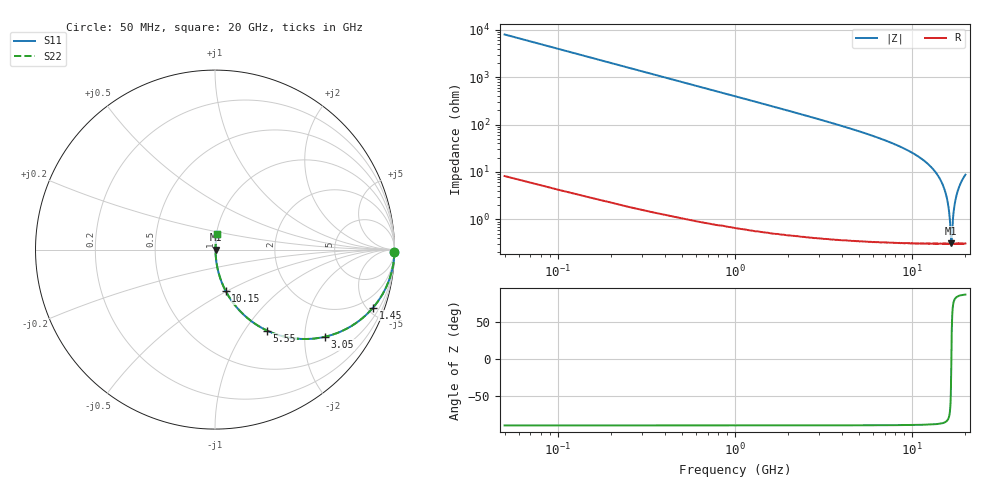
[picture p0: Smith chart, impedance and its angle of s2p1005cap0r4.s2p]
!	AVX	Thin	Film	Operation
!	Date:	March 2012
!	Description: Ultra-Miniature 01005 Size ACCU - P® Thin Film RF / Microwave Capacitor
!	Part Number:  C005YJ0R4ABSTR
!	Serial	Measurements
#	MHz	S	db	R	50
!	S11	S21	S12	S22
!	dB	Phase	dB	Phase	dB	Phase	dB	Phase
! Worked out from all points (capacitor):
!   400 points, 50 MHz to 20 GHz, reference 50 ohm
!   read as one part in series: C = 400 fF near 150 MHz
!   lowest |Z| = 312 mohm at 16.65 GHz (marker M1)
!   series resonance near 16.67 GHz, so ESL is about 230 pH
!   S11 on the Smith chart (normalised r, x): 50 MHz: open; 1.45 GHz: 1.01, -5.45; 3.05 GHz: 1.01, -2.52; 5.55 GHz: 1.01, -1.27; 10.15 GHz: 1.01, -0.49; 20 GHz: 1.01, +0.18
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50  -0.00 -0.7  -38.02 89.2  -38.02 89.2  -0.00 -0.7
100  -0.00 -1.4  -32.00 88.5  -32.00 88.5  -0.00 -1.4
150  -0.01 -2.2  -28.48 87.8  -28.48 87.8  -0.01 -2.2
400  -0.04 -5.7  -19.99 84.2  -19.99 84.2  -0.04 -5.7
800  -0.17 -11.4  -14.09 78.5  -14.09 78.5  -0.17 -11.4
1450  -0.56 -20.1  -9.26 69.7  -9.26 69.7  -0.56 -20.1
3050  -2.13 -38.3  -4.15 51.5  -4.15 51.5  -2.13 -38.3
3400  -2.56 -41.6  -3.55 48.2  -3.55 48.2  -2.56 -41.6
5550  -5.41 -57.3  -1.50 32.4  -1.50 32.4  -5.41 -57.3
6700  -7.04 -63.2  -0.98 26.4  -0.98 26.4  -7.04 -63.2
10050  -12.27 -75.2  -0.29 14.1  -0.29 14.1  -12.27 -75.2
10150  -12.44 -75.5  -0.28 13.8  -0.28 13.8  -12.44 -75.5
13350  -19.50 -82.3  -0.08 6.1  -0.08 6.1  -19.50 -82.3
14750  -24.69 -83.7  -0.04 3.3  -0.04 3.3  -24.69 -83.7
15700  -30.88 -82.2  -0.03 1.6  -0.03 1.6  -30.88 -82.2
16250  -38.13 -75.1  -0.03 0.7  -0.03 0.7  -38.13 -75.1
16650  -50.23 -8.3  -0.03 0.0  -0.03 0.0  -50.23 -8.3
16700  -49.89 17.8  -0.03 -0.1  -0.03 -0.1  -49.89 17.8
17050  -38.96 73.7  -0.03 -0.6  -0.03 -0.6  -38.96 73.7
17650  -31.22 82.1  -0.03 -1.6  -0.03 -1.6  -31.22 82.1
18600  -25.61 83.7  -0.04 -3.0  -0.04 -3.0  -25.61 83.7
20000  -21.21 83.0  -0.06 -5.0  -0.06 -5.0  -21.21 83.0
